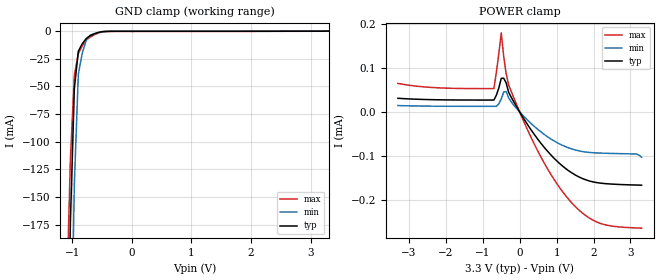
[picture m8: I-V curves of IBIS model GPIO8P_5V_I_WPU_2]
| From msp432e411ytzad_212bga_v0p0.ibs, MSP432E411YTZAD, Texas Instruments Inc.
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|   Model Cell GPIO8P_5V_I_WPU_2
[Model]   GPIO8P_5V_I_WPU_2
Model_type   Input
Polarity   Non-Inverting
Vinl =  0.8
Vinh =  2
C_comp   7.738177p   6.063161p   9.392973p
[Model Spec]
Vinl   0.8   0.8   0.8
Vinh   2   2   2
[Temperature Range]   25   125   -40
[Voltage Range]   3.3   2.97   3.63
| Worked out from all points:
|   GND clamp passes 1 mA (typ) near -0.54 V on its own axis
| Nom Voltages:
|   VDDC=1.2, VDD=3.3, GND=0
| Min Voltages:
|   VDDC=1.08, VDD=2.97, GND=0
| Max Voltages:
|   VDDC=1.32, VDD=3.63, GND=0
[POWER_clamp]
|   voltage   I(typ)   I(min)   I(max)
-3.3V     31.22uA    14.77uA    64.95uA
-700mV    27.24uA    13.03uA    53.12uA
-500mV    76.46uA    29.87uA    179.4uA
-433.3mV  76.57uA    45.65uA    125.7uA
-366.7mV  65.99uA    46.46uA    86.4uA
-300mV    44.74uA    32.31uA    61.57uA
433.3mV   -55.14uA   -35.25uA   -78.95uA
1.1V      -118uA     -73.05uA   -173.5uA
1.567V    -145.3uA   -87.19uA   -219uA
2.033V    -159uA     -92.33uA   -246.9uA
3.167V    -165.3uA   -95.12uA   -262.6uA
3.3V      -165.6uA   -102.3uA   -263uA
[GND_clamp]
|   voltage   I(typ)   I(min)   I(max)
-3.3V     -16.36A    -15.34A    -17.18A
-1.1V     -382.1mA   -633.4mA   -250.1mA
-1.033V   -173.3mA   -336.5mA   -116.4mA
-966.7mV  -52.02mA   -138.4mA   -39.81mA
-900mV    -18.21mA   -38.99mA   -20.35mA
-833.3mV  -11.38mA   -19.83mA   -13.21mA
-766.7mV  -6.658mA   -8.069mA   -8.223mA
-700mV    -4.058mA   -3.706mA   -5.385mA
-500mV    -482.9uA   -471.4uA   -624.5uA
-366.7mV  -181.5uA   -126.7uA   -278.7uA
3.3V      692.5pA    38.99uA    -61.41uA
